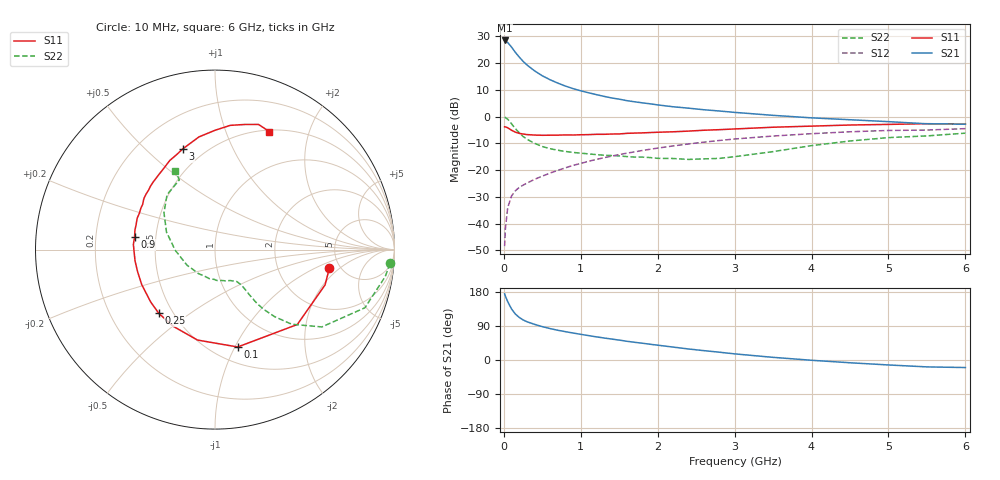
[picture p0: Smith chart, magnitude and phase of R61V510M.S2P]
! SIEMENS Small Signal Semiconductors
! BFR193
! Si NPN RF Bipolar Junction Transistor in SOT23
! VCE = 1.5 V  IC = 10 mA
! Common Emitter S-Parameters:  May  1996
# GHz  S  MA  R  50
!  f  S11  S21  S12  S22
! GHz  MAG  ANG  MAG  ANG  MAG  ANG  MAG  ANG
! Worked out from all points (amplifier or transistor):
!   36 points, 10 MHz to 6 GHz, reference 50 ohm
!   highest |S21| = 28.5 dB at 10 MHz (marker M1)
!   |S21| within 3 dB of that: start of sweep to 113.3 MHz
!   unconditionally stable (mu >= 1): 695.2 MHz to 2.036 GHz
!   at 250 MHz: K = 0.65, MSG = 23.1 dB, |S12| = -25.6 dB
!   at 1.4 GHz: K = 1.05, MAG = 9.6 dB, |S12| = -14.8 dB
!   at 6 GHz: K = 0.96, MSG = 0.8 dB, |S12| = -4.5 dB
!   S11 on the Smith chart (normalised r, x): 10 MHz: 4.11, -1.44; 100 MHz: 0.65, -1.03; 250 MHz: 0.42, -0.38; 900 MHz: 0.38, +0.07; 3 GHz: 0.38, +0.66; 6 GHz: 0.52, +1.43
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0.01  0.6458 -9.1  26.51 174.6  0.0038 88.1  0.9792 -4.5
0.02  0.644 -17.8  26.07 168.9  0.008 81.4  0.9603 -9.0
0.05  0.62 -42.3  24.34 154.1  0.0199 72.6  0.896 -21.2
0.1  0.5571 -76.9  19.96 134.6  0.0329 61.6  0.7348 -35.9
0.15  0.5133 -101.0  15.84 121.2  0.0413 55.6  0.5967 -44.2
0.2  0.4866 -118.5  12.98 112.4  0.0475 53.9  0.4992 -48.4
0.25  0.4735 -131.4  10.82 105.8  0.0525 54.0  0.4267 -50.9
0.3  0.4622 -140.8  9.244 101.0  0.0573 55.1  0.3783 -52.1
0.4  0.4525 -154.4  7.164 94.0  0.0674 56.5  0.3171 -52.7
0.5  0.4485 -164.1  5.796 88.0  0.0774 58.5  0.2766 -52.9
0.6  0.4499 -172.1  4.899 83.0  0.088 60.0  0.2518 -53.3
0.7  0.451 -178.8  4.238 78.6  0.0991 61.0  0.2361 -54.0
0.9  0.4535 171.1  3.337 71.2  0.1227 61.7  0.2145 -55.9
1.1  0.4612 162.3  2.795 64.4  0.1463 61.7  0.2015 -60.2
1.3  0.4674 154.5  2.396 58.1  0.1707 60.7  0.1901 -64.9
1.6  0.4875 144.4  1.989 49.4  0.2078 58.5  0.1791 -74.8
2.2  0.5211 127.2  1.529 34.1  0.2835 52.2  0.1651 -100.9
3  0.5886 107.9  1.201 16.2  0.382 40.9  0.1785 -150.7
3.5  0.6342 98.1  1.057 7.0  0.434 33.1  0.222 -179.2
4.5  0.6974 83.0  0.875 -7.3  0.5214 18.1  0.3509 144.1
5.5  0.7382 70.8  0.735 -18.2  0.5616 3.1  0.4364 117.1
6  0.7242 65.3  0.725 -19.9  0.597 -1.4  0.4913 116.7
